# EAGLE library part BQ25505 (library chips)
EH front end for switching between primary and secondary cells
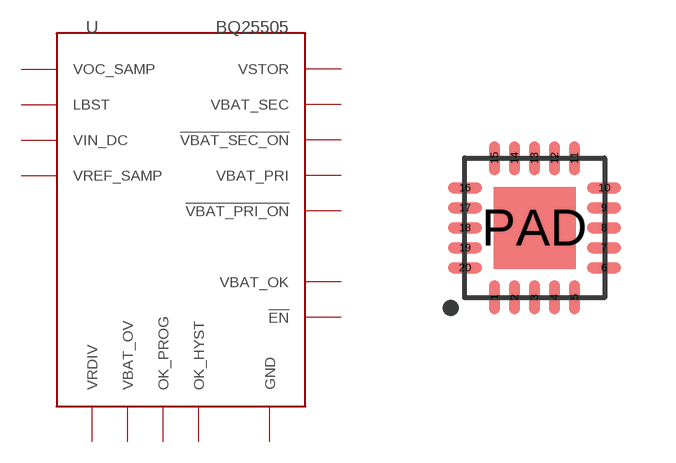
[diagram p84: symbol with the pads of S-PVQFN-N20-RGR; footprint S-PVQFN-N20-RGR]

Designator prefix U

## BQ25505 (DIGIKEY: 296-37078-1-ND; MANUFACTURER: TI; MPN: BQ25505RGRR)  [S-PVQFN-N20-RGR]
1  GND
2  VIN_DC
3  VOC_SAMP
4  VREF_SAMP
5  !EN
6  GND
7  VBAT_OV
8  VRDIV
9  !VBAT_SEC_ON
10  !VBAT_PRI_ON
11  OK_HYST
12  OK_PROG
13  VBAT_OK
14  VBAT_PRI
15  GND
16  GND
17  GND
18  VBAT_SEC
19  VSTOR
20  LBST
PAD  GND

## Footprint S-PVQFN-N20-RGR (pad centres in mm)
smd 0.28 x 0.85: 1 -1,-1.74; 2 -0.5,-1.74; 3 0,-1.74; 4 0.5,-1.74; 5 1,-1.74; 11 1,1.74; 12 0.5,1.74; 13 0,1.74; 14 -0.5,1.74; 15 -1,1.74
smd 0.85 x 0.28: 6 1.74,-1; 7 1.74,-0.5; 8 1.74,0; 9 1.74,0.5; 10 1.74,1; 16 -1.74,1; 17 -1.74,0.5; 18 -1.74,0; 19 -1.74,-0.5; 20 -1.74,-1
smd 2.05 x 2.05: PAD 0,0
